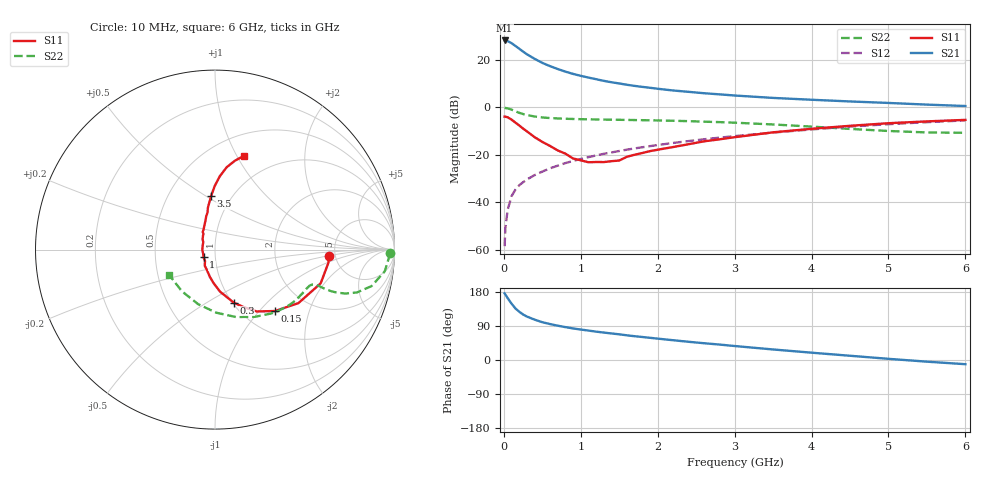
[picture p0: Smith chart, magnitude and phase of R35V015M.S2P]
! SIEMENS Small Signal Semiconductors
! BFR181
! Si NPN RF Bipolar Junction Transistor in SOT23
! VCE = 5 V  IC = 15 mA
! Common Emitter S-Parameters:  May  1996
# GHz  S  MA  R  50
!  f  S11  S21  S12  S22
! GHz  MAG  ANG  MAG  ANG  MAG  ANG  MAG  ANG
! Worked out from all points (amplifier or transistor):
!   36 points, 10 MHz to 6 GHz, reference 50 ohm
!   highest |S21| = 28.2 dB at 10 MHz (marker M1)
!   |S21| within 3 dB of that: start of sweep to 179.9 MHz
!   unconditionally stable (mu >= 1): 650.8 MHz to 2.559 GHz
!   at 250 MHz: K = 0.71, MSG = 27.5 dB, |S12| = -31.5 dB
!   at 1.4 GHz: K = 1.06, MAG = 13.2 dB, |S12| = -19.0 dB
!   at 6 GHz: K = 0.85, MSG = 3.0 dB, |S12| = -5.5 dB
!   S11 on the Smith chart (normalised r, x): 10 MHz: 4.45, -0.57; 150 MHz: 1.38, -1.22; 300 MHz: 1.01, -0.66; 1 GHz: 0.88, -0.08; 3.5 GHz: 0.80, +0.53; 6 GHz: 0.72, +1.07
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0.01  0.6379 -3.4  25.56 175.9  0.0012 95.6  0.9767 -1.2
0.02  0.6357 -6.8  25.25 172.6  0.0029 80.2  0.9691 -2.9
0.05  0.6181 -17.7  24.74 163.2  0.007 80.1  0.9535 -7.3
0.1  0.5522 -32.7  22.43 148.8  0.0135 78.3  0.8958 -13.1
0.15  0.4781 -45.7  19.62 136.2  0.0185 72.2  0.8262 -16.8
0.2  0.4157 -56.0  17.14 127.4  0.0229 70.8  0.7679 -18.6
0.25  0.3579 -63.5  14.89 120.1  0.0266 69.8  0.723 -19.4
0.3  0.3127 -70.6  13.1 114.6  0.0304 70.3  0.6883 -19.7
0.4  0.2361 -83.1  10.49 106.5  0.0375 71.0  0.6423 -19.6
0.5  0.1875 -92.3  8.627 99.7  0.0445 71.7  0.6135 -19.3
0.6  0.1543 -100.7  7.368 94.9  0.0521 72.1  0.5958 -19.3
0.7  0.1242 -110.8  6.413 90.5  0.0593 72.8  0.5839 -19.5
0.8  0.1062 -122.3  5.646 86.8  0.0672 72.2  0.5752 -19.8
1  0.0769 -146.4  4.602 80.3  0.0821 72.7  0.5636 -20.9
1.1  0.0699 -160.9  4.232 77.7  0.0897 72.5  0.5599 -21.8
1.3  0.0706 170.5  3.608 72.4  0.1054 71.7  0.5527 -23.6
1.6  0.0913 139.2  2.987 65.1  0.1288 70.3  0.5442 -26.9
2.2  0.1461 113.8  2.265 52.2  0.1782 66.8  0.5221 -35.0
3.5  0.2983 94.2  1.58 27.8  0.2947 55.7  0.4365 -59.0
4.5  0.409 86.3  1.331 11.2  0.3936 44.5  0.3517 -88.8
5.5  0.5065 77.5  1.142 -4.4  0.4879 31.5  0.2966 -128.5
6  0.5452 73.0  1.067 -11.1  0.5311 24.3  0.2914 -150.7
